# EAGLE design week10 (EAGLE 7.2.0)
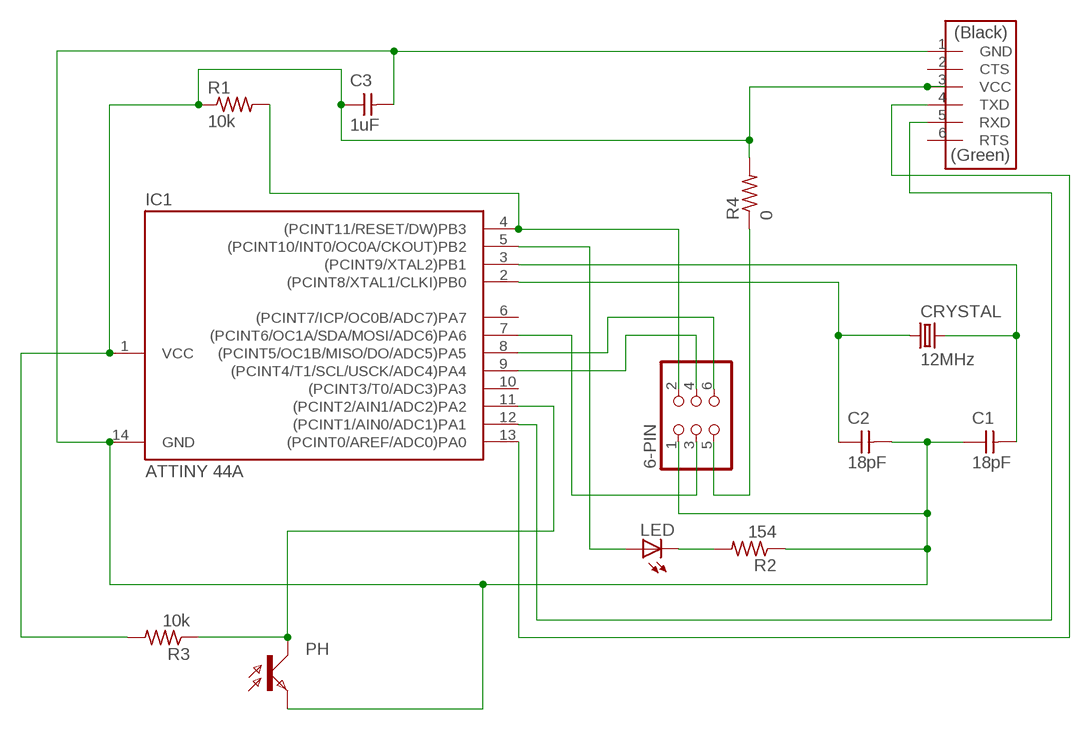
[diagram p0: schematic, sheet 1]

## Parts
6-PIN  PINHD-2X3-SMD  [2X03SMD]
C1  18pF  CAP-UNPOLARIZEDFAB  [C1206FAB]
C2  18pF  CAP-UNPOLARIZEDFAB  [C1206FAB]
C3  1uF  CAP-UNPOLARIZEDFAB  [C1206FAB]
CRYSTAL  12MHz  CRYSTAL-120ECSR  [CRYSTAL-120ECSR]
FTDI  FTDI-HEADER  FTDI-SMD-HEADER  [1X06SMD]
IC1  ATTINY 44A  ATTINY44-SSU  [SOIC14]
LED  LED  [LED1206]
PH  PHOTOTRANSISTOR-NPN1206  [OP1206]
R1  10k  RES-US1206FAB  [R1206FAB]
R2  154  RES-US1206FAB  [R1206FAB]
R3  10k  RES-US1206FAB  [R1206FAB]
R4  0  RES-US1206FAB  [R1206FAB]

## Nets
_: 6-PIN.3 IC1.7((PCINT6/OC1A/SDA/MOSI/ADC6)PA6)
N$2: 6-PIN.1 C1.1 C2.2 C3.2 FTDI.1(GND) IC1.14(GND) PH.EMITTER(E) R2.1
N$3: C2.1 CRYSTAL.P$1 IC1.2((PCINT8/XTAL1/CLKI)PB0)
N$4: C1.2 CRYSTAL.P$2 IC1.3((PCINT9/XTAL2)PB1)
N$5: IC1.5((PCINT10/INT0/OC0A/CKOUT)PB2) LED.1(A)
N$6: LED.2(C) R2.2
N$7: FTDI.4(TXD) IC1.13((PCINT0/AREF/ADC0)PA0)
N$8: FTDI.5(RXD) IC1.12((PCINT1/AIN0/ADC1)PA1)
N$9: C3.1 FTDI.3(VCC) IC1.1(VCC) R1.1 R3.2 R4.2
N$10: IC1.11((PCINT2/AIN1/ADC2)PA2) PH.COLLECTOR(C) R3.1
N$11: 6-PIN.2 IC1.4((PCINT11/RESET/DW)PB3) R1.2
N$12: 6-PIN.4 IC1.9((PCINT4/T1/SCL/USCK/ADC4)PA4)
N$13: 6-PIN.6 IC1.8((PCINT5/OC1B/MISO/DO/ADC5)PA5)
N$14: 6-PIN.5 R4.1
Unconnected: FTDI.2(CTS) FTDI.6(RTS) IC1.6((PCINT7/ICP/OC0B/ADC7)PA7) IC1.10((PCINT3/T0/ADC3)PA3)

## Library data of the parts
6-PIN = fab:PINHD-2X3-SMD: PIN HEADER
C1-C3 = fab:CAP-UNPOLARIZED
CRYSTAL = fab:CRYSTAL-120ECSR
FTDI = fab:FTDI-SMD-HEADER
IC1 = fab:ATTINY44
LED = fab:LED: LED
PH = fab:PHOTOTRANSISTOR-NPN
R1-R4 = fab:RES-US: Resistor (US Symbol)

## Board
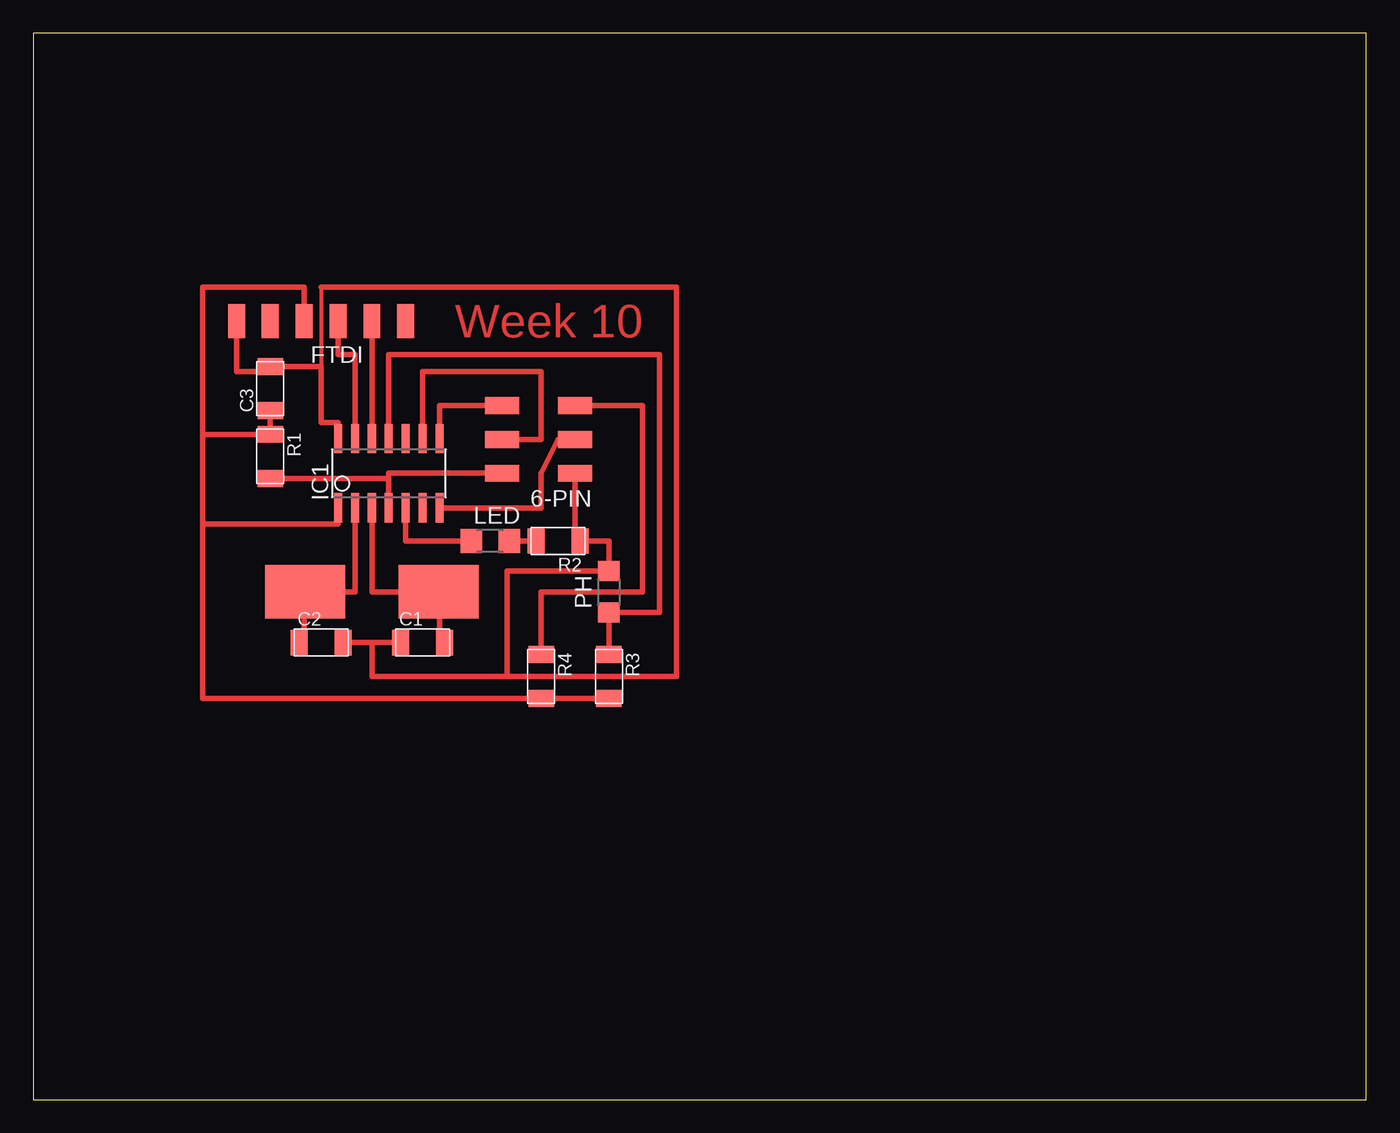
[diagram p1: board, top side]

Size 100 x 80 mm. Coordinates in mm from the lower left corner, seen from the top.
Outline: 0,0 100,0 100,80 0,80 0,0
Copper layers (1*16): Top 0.035mm / dielectric 1.5mm / Bottom 0.035mm
Design rules "default *": minimum track width 10mil, minimum drill 24mil, track to track 18mil, track to pad 18mil, pad to pad 18mil, via to via 18mil, smd to smd 8mil, copper to edge 40mil, drill to drill 8mil, minimum pad ring 10mil, minimum via ring 8mil, stop-mask expansion 4mil, vias tented up to drill 0mil, thermal gap 10mil

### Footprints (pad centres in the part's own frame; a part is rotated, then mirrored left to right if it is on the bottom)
2X03SMD = smd 2.54 x 1.27: 1 -2.54,2.54; 2 2.92,2.54; 3 -2.54,0; 4 2.92,0; 5 -2.54,-2.54; 6 2.92,-2.54
C1206FAB = smd 1.27 x 1.905: 1 -1.651,0; 2 1.651,0
CRYSTAL-120ECSR = smd 6 x 4: P$1 -5,0; P$2 5,0
1X06SMD = smd 2.54 x 1.27: 1 0,6.35; 2 0,3.81; 3 0,1.27; 4 0,-1.27; 5 0,-3.81; 6 0,-6.35
SOIC14 = smd 0.61 x 2.21: 1 -3.81,-2.603; 2 -2.54,-2.603; 3 -1.27,-2.603; 4 0,-2.603; 5 1.27,-2.603; 6 2.54,-2.603; 7 3.81,-2.603; 8 3.81,2.603; 9 2.54,2.603; 10 1.27,2.603; 11 0,2.603; 12 -1.27,2.603; 13 -2.54,2.603; 14 -3.81,2.603
LED1206 = smd 1.6 x 1.803: 1 -1.422,0; 2 1.422,0
OP1206 = smd 1.5 x 1.6: COLLECTOR -1.55,0; EMITTER 1.55,0
R1206FAB = smd 1.27 x 1.905: 1 -1.651,0; 2 1.651,0

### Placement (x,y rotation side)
6-PIN  38.1,49.53 180 top
C1  29.21,34.29 0 top
C2  21.59,34.29 0 top
C3  17.78,53.34 90 top
CRYSTAL  25.4,38.1 0 top
FTDI  21.59,58.42 90 top
IC1  26.67,46.99 0 top
LED  34.29,41.91 0 top
PH  43.18,38.1 90 top
R1  17.78,48.26 270 top
R2  39.37,41.91 180 top
R3  43.18,31.75 270 top
R4  38.1,31.75 270 top

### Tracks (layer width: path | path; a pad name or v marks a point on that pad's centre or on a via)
_
  Top 0.406: IC1.7 38.1,44.39 38.1,46.99 39.37,49.53 6-PIN.3
N$2
  Top 0.305: 21.59,60.96 21.59,54.99
  Top 0.406: 6-PIN.1 40.64,41.91 R2.1 43.18,41.91 PH.EMITTER 35.56,39.65 35.56,31.75 | C2.2 25.4,34.29 | 25.4,34.29 C1.1 | 35.56,31.75 25.4,31.75 25.4,34.29 | FTDI.1 15.24,54.61 17.78,54.61 C3.2 21.59,54.99 21.59,50.8 22.86,50.8 IC1.14 | 35.56,31.75 48.26,31.75 48.26,60.96 21.59,60.96
N$3
  Top 0.406: C2.1 20.32,34.29 20.32,36.83 20.4,36.83 CRYSTAL.P$1 24.13,38.1 IC1.2
N$4
  Top 0.406: IC1.3 25.4,38.1 CRYSTAL.P$2 30.48,38.1 30.48,34.29 C1.2
N$5
  Top 0.406: LED.1 27.94,41.91 IC1.5
N$6
  Top 0.406: LED.2 R2.2
N$7
  Top 0.406: FTDI.4 22.86,55.88 24.13,55.88 IC1.13
N$8
  Top 0.406: FTDI.5 IC1.12
N$9
  Top 0.406: R3.2 R4.2 12.7,30.1 12.7,43.18 | 12.7,43.18 22.86,43.18 IC1.1 | 12.7,49.91 12.7,60.96 20.32,60.96 FTDI.3 | 12.7,49.91 12.7,43.18 | C3.1 R1.1 12.7,49.91
N$10
  Top 0.406: R3.1 PH.COLLECTOR 46.99,36.55 46.99,55.88 26.67,55.88 IC1.11
N$11
  Top 0.406: R1.2 26.67,46.61 IC1.4 26.67,46.99 6-PIN.2
N$12
  Top 0.406: IC1.9 29.21,54.61 38.1,54.61 38.1,49.53 6-PIN.4
N$13
  Top 0.406: 6-PIN.6 30.48,52.07 IC1.8 30.48,49.53
N$14
  Top 0.406: R4.1 38.1,38.1 45.72,38.1 45.72,52.07 6-PIN.5

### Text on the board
Top: Week 10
